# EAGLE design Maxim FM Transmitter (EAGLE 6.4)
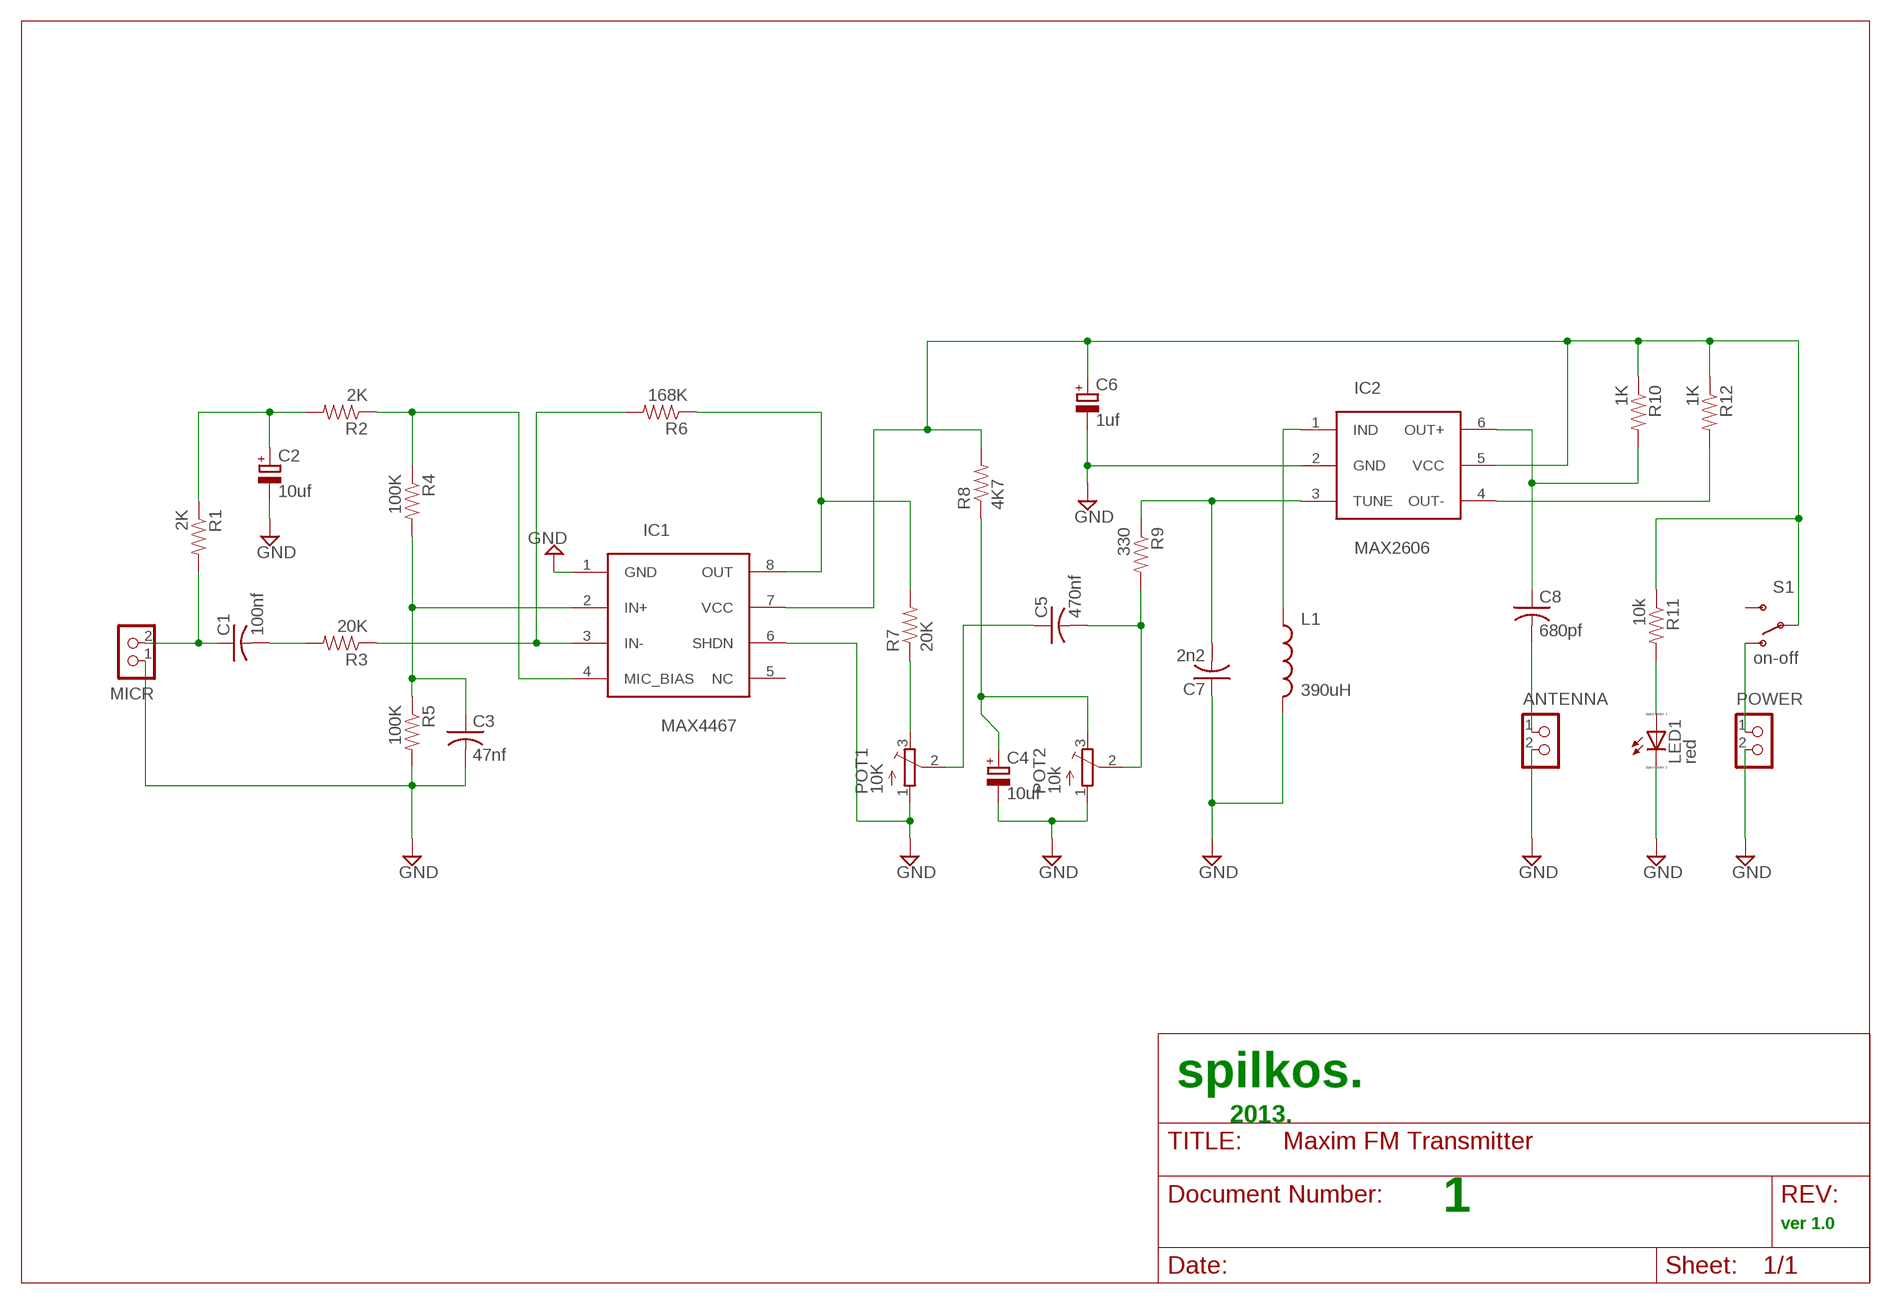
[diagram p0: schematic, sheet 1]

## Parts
ANTENNA  CON_HEADER_1X02-PTH  [M1X2]
C1  100nf  C-USC0805  [C0805]
C2  10uf  CPOL-EUSANYO_SMD_A5  [SANYO-OSCON_SMD_A5]
C3  47nf  C-USC0805  [C0805]
C4  10uf  CPOL-EUSANYO_SMD_A5  [SANYO-OSCON_SMD_A5]
C5  470nf  C-USC0805  [C0805]
C6  1uf  CPOL-EUSANYO_SMD_A5  [SANYO-OSCON_SMD_A5]
C7  2n2  C-USC0805  [C0805]
C8  680pf  C-USC0805  [C0805]
IC1  MAX4467  MAX4467-SOT-23-8L  [MAX4467-SOT-23-8L]
IC2  MAX2606  MAX2606-SOT-23-6L  [MAX2606-SOT-23-6L]
L1  390uH  INDUCTOR0805  [0805]
LED1  red  LED_ESML0603  [LED_SML0603]
MICR  micr  CON_HEADER_1X02-PTH  [M1X2]
POT1  10K  TRIMPOTTC33X  [TC33X]
POT2  10k  TRIMPOTTC33X  [TC33X]
POWER  power  CON_HEADER_1X02-PTH  [M1X2]
R1  2K  RESISTOR0805-RES  [0805]
R2  2K  RESISTOR0805-RES  [0805]
R3  20K  RESISTOR0805-RES  [0805]
R4  100K  RESISTOR0805-RES  [0805]
R5  100K  RESISTOR0805-RES  [0805]
R6  168K  RESISTOR0805-RES  [0805]
R7  20K  RESISTOR0805-RES  [0805]
R8  4K7  RESISTOR0805-RES  [0805]
R9  330  RESISTOR0805-RES  [0805]
R10  1K  RESISTOR0805-RES  [0805]
R11  10k  RESISTOR0805-RES  [0805]
R12  1K  RESISTOR0805-RES  [0805]
S1  on-off  SWITCH-SPDTSMD2  [SWITCH-SPDT-SMD]

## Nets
GND: ANTENNA.2 C2.- C3.2 C4.- C6.- C7.1 IC1.1(GND) IC1.6(SHDN) IC2.2(GND) L1.2 LED1.C MICR.1 POT1.1(A) POT2.1(A) POWER.2 R5.2
N$1: C1.1 MICR.2 R1.2
N$2: C1.2 R3.2
N$3: IC1.3(IN-) R3.1 R6.2
N$4: POT1.3(E) R7.1
N$5: C2.+ R1.1 R2.2
N$6: IC1.4(MIC_BIAS) R2.1 R4.1
N$7: C3.1 IC1.2(IN+) R4.2 R5.1
N$8: IC1.8(OUT) R6.1 R7.2
N$9: C4.+ POT2.3(E) R8.1
N$10: LED1.A R11.2
N$11: C5.1 POT1.2(S)
N$12: C5.2 POT2.2(S) R9.2
N$13: C7.2 IC2.3(TUNE) R9.1
N$14: IC2.1(IND) L1.1
N$15: IC2.4(OUT-) R12.2
N$16: ANTENNA.1 C8.2
N$17: C8.1 IC2.6(OUT+) R10.2
N$18: POWER.1 S1.1(O)
POWER: C6.+ IC1.7(VCC) IC2.5(VCC) R8.2 R10.1 R11.1 R12.1 S1.2(P)
Unconnected: IC1.5(NC) S1.3(S)

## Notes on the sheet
- spilkos.
- 2013.
- 1
- ver 1.0

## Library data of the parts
ANTENNA MICR POWER = dp_devices:CON_HEADER_1X02
C1 C3 C5 C7 C8 = adafruit:C-US: CAPACITOR, American symbol
C2 C4 C6 = rcl:CPOL-EU: POLARIZED CAPACITOR, European symbol
IC1 = MAX4467:MAX4467-SOT-23-8L
IC2 = MAX2606:MAX2606-SOT-23-6L
L1 = SparkFun-Passives:INDUCTOR: Inductors
LED1 = eagle-ltspice:LED_E: LED; SPICEMODEL: NONE; SPICEPREFIX: D; SPICETYPE: diode
POT1 POT2 = adafruit:TRIMPOT: SMT trimmer potentiometer part number TC33X http://www.ladyada.net/library/eagle
R1-R12 = SparkFun-Passives:RESISTOR: Resistor
S1 = SparkFun-Electromechanical:SWITCH-SPDT: SPDT Switch Simple slide switch, Spark Fun Electronics SKU : COM-00102 DPDT SMT slide switch, AYZ0202, SWCH-08179

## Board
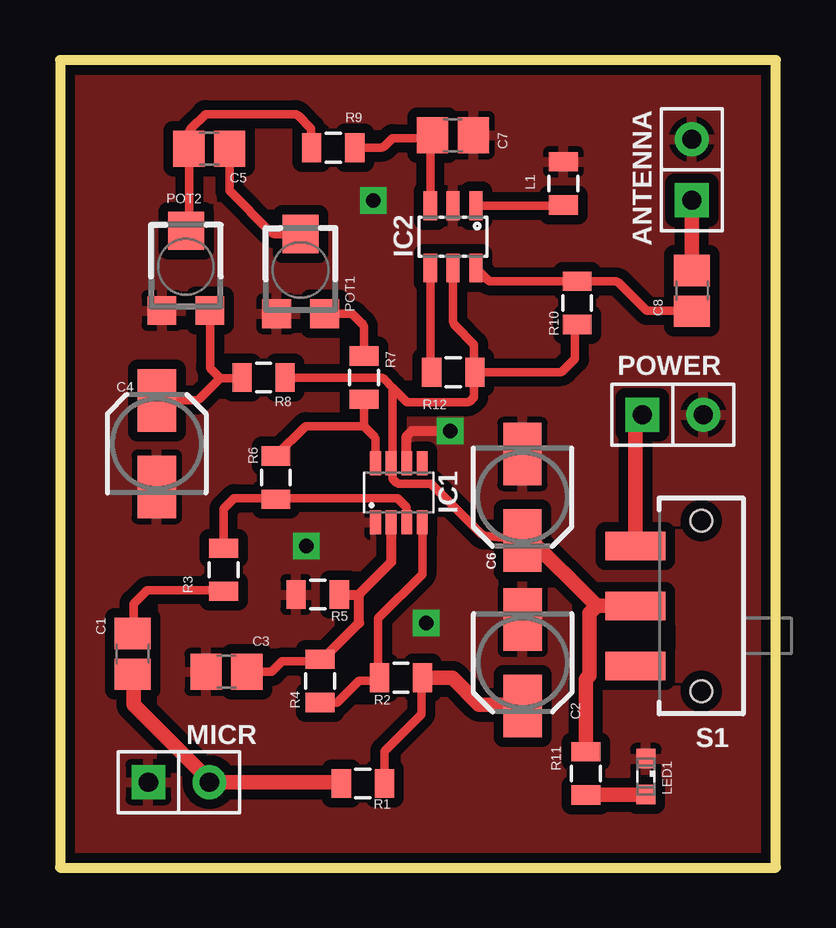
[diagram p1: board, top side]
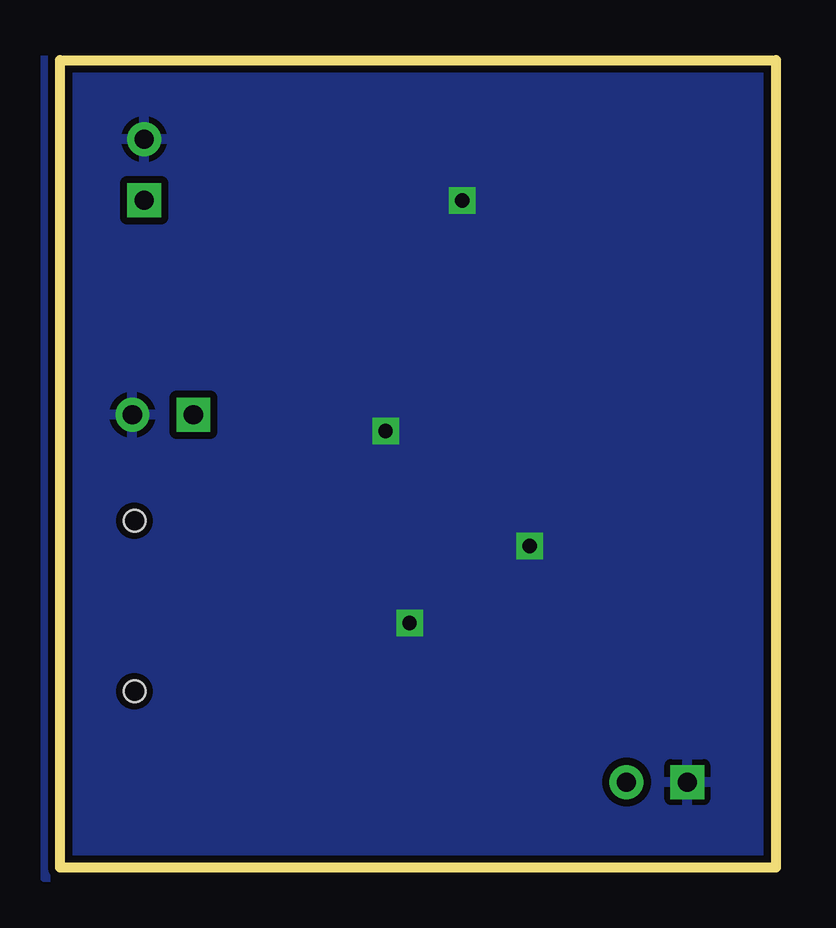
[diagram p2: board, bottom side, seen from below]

Size 29.84 x 33.66 mm. Coordinates in mm from the lower left corner, seen from the top.
Outline: 29.84,33.66 0,33.66 0,0 29.84,0 29.84,33.66
Copper layers (1*16): Top 0.035mm / dielectric 1.5mm / Bottom 0.035mm
Design rules "SparkFun": minimum track width 8mil, minimum drill 20mil, track to track 8mil, track to pad 8mil, pad to pad 8mil, via to via 8mil, smd to smd 8mil, copper to edge 10mil, drill to drill 8mil, minimum pad ring 12mil, minimum via ring 10mil, stop-mask expansion 4mil, vias tented up to drill 25mil, thermal gap 10mil
tRestrict: area 22.3,9.2 to 25.3,10; area 12.3,7.2 to 13.1,10.2; area 10.1,16 to 12.5,17.8

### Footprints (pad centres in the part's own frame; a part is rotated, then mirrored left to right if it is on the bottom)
M1X2 = drill 0.8 square: 1 -1.27,0 | drill 0.8: 2 1.27,0
C0805 = smd 1.3 x 1.5: 1 -0.85,0; 2 0.85,0
SANYO-OSCON_SMD_A5 = smd 2.6 x 1.6: + 1.8,0; - -1.8,0
MAX4467-SOT-23-8L = smd 1 x 0.45: 1 -1.225,0.975; 2 -1.225,0.325; 3 -1.225,-0.325; 4 -1.225,-0.975; 5 1.225,-0.975; 6 1.225,-0.325; 7 1.225,0.325; 8 1.225,0.975
MAX2606-SOT-23-6L = smd 1.2 x 0.55: 1 -1.3,0.95; 2 -1.3,0; 3 -1.3,-0.95; 4 1.3,-0.95; 5 1.3,0; 6 1.3,0.95
0805 = smd 0.8 x 1.2: 1 -0.9,0; 2 0.9,0
LED_SML0603 = smd 0.8 x 0.8: A 0.75,0; C -0.75,0
TC33X = smd 1.2 x 1.2: 1 -1,-1.825; 3 1,-1.825 | smd 1.5 x 1.6: 2 0,1.5
SWITCH-SPDT-SMD = smd 1.2 x 2.5: 1 -2.5,-2.75; 2 0,-2.75; 3 2.5,-2.75 | hole 0.9: -3.55,0; 3.55,0

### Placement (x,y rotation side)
ANTENNA  26.34,29.08 90 top
C1  3.03,8.91 90 top
C2  19.29,8.54 270 top
C3  6.95,8.16 180 top
C4  4.04,17.67 90 top
C5  6.23,29.96 180 top
C6  19.28,15.44 270 top
C7  16.38,30.52 180 top
C8  26.35,24.04 90 top
IC1  14.13,15.63 90 top
IC2  16.39,26.29 270 top
L1  20.99,28.51 90 top
LED1  24.43,3.8 270 top
MICR  4.96,3.57 0 top
POT1  10.03,24.9 0 top
POT2  5.25,25.04 0 top
POWER  25.55,18.88 0 top
R1  12.63,3.51 180 top
R2  14.22,7.91 0 top
R3  6.82,12.42 270 top
R4  10.85,7.78 90 top
R5  10.74,11.38 180 top
R6  9,16.26 270 top
R7  12.67,20.42 270 top
R8  8.49,20.42 0 top
R9  11.39,30 180 top
R10  21.56,23.53 90 top
R11  21.93,3.93 270 top
R12  16.4,20.65 180 top
S1  26.74,10.91 270 top

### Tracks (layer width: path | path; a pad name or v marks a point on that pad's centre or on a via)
GND  (via drill 0.6)
  Top 0.406: IC1.6 14.46,17.99 14.67,18.2 v16.27,18.2
  other vias: 13.07,27.8 15.27,10.2 10.27,13.4
  pour Top (isolate 0.406): 0,33.97 30.16,33.97 30.16,-0.32 0,-0.32
  pour Bottom (isolate 0.305): -0.33,34 30.22,34 30.47,33.75 30.47,-0.4 -0.08,-0.4 -0.33,-0.15
N$1
  Top 0.61: R1.2 11.67,3.57 MICR.2 6.23,3.64 3.07,6.8 3.07,8.02 C1.1
N$2
  Top 0.35: R3.2 6.78,11.56 3.63,11.56 3.07,11 3.07,9.79 C1.2
N$3
  Top 0.35: IC1.3 14.46,15.01 14.07,15.4 9.04,15.4 R6.2 8.96,15.4 7.27,15.4 6.82,14.95 R3.1
N$4
  Top 0.35: R7.1 12.67,22.49 arc45 12.6,22.67 12.26,23 arc45 12.09,23.08 POT1.3
N$5
  Top 0.35: R1.1 13.53,4.86 15.07,6.4 15.07,7.86 R2.2
  Top 0.61: R2.2 16.36,7.91 17.47,6.8 18.83,6.8 C2.+
N$6
  Top 0.35: IC1.4 15.11,12.24 13.27,10.4 13.27,7.96 R2.1 13.21,7.8 12.47,7.8 11.55,6.88 R4.1
N$7
  Top 0.35: 10.84,8.69 arc45 R4.2 | 10.75,8.72 arc-45 R4.2 | C3.1 8.83,8.16 9.27,8.6 10.76,8.6 R4.2
  Top 0.406: IC1.2 13.81,12.74 12.45,11.38 | R5.1 12.45,11.38 | R4.2 10.95,8.68 12.47,10.2 12.47,11.36 12.45,11.38
N$8
  Top 0.35: IC1.8 13.16,17.81 arc45 13.08,17.99 12.67,18.4 | 12.67,18.4 R7.2 arc-45 R7.2 | R6.1 10.24,18.4 12.67,18.4
N$9
  Top 0.35: POT2.3 6.25,20.93 arc45 6.32,20.75 6.67,20.4 | 6.67,20.4 7.53,20.4 arc45 R8.1 | C4.+ 5.63,19.47 arc45 5.81,19.54 6.67,20.4
N$10
  Top 0.61: R11.2 24.41,3.03 LED1.A
N$11
  Top 0.35: POT1.2 8.97,26.4 arc-45 8.79,26.48 7.07,28.2 7.07,29.94 arc-45 C5.1
N$12
  Top 0.35: POT2.2 5.3,26.79 arc45 5.38,26.97 C5.2 5.38,30.6 arc-45 5.45,30.78 6.07,31.4 9.76,31.4 arc-45 9.94,31.33 10.47,30.8 10.47,30.05 arc45 R9.2
N$13
  Top 0.35: R9.1 13.37,30 arc45 13.55,30.08 13.87,30.4 15.3,30.4 arc45 15.48,30.47 C7.2 15.51,30.5 arc45 15.44,30.32 IC2.3
N$14
  Top 0.35: IC2.1 20.97,27.59 L1.1
N$15
  Top 0.35: IC2.4 15.44,20.79 arc45 R12.2
N$16
  Top 0.61: C8.2 26.35,27.78 arc45 ANTENNA.1
N$17
  Top 0.35: IC2.6 17.82,24.5 arc45 18,24.43 R10.2 23.13,24.43 arc-45 23.31,24.36 24.47,23.2 26.32,23.2 arc-45 C8.1
N$18
  Top 0.61: POWER.1 24.24,18.88 arc90 23.99,18.62 S1.1
POWER
  Top 0.35: R12.1 20.81,20.65 arc45 20.99,20.72 21.47,21.2 21.47,22.43 arc-45 21.54,22.61 R10.1 | IC2.5 16.39,22.79 arc45 16.46,22.61 17.27,21.8 17.27,20.71 arc45 R12.1 | C6.+ 17.73,13.84 arc-45 17.55,13.91 15.47,16 14.17,16 arc-45 14,16.07 13.87,16.2 13.87,16.7 arc45 IC1.7 arc45 13.87,17 13.87,20 | R8.2 13.34,20.42 arc-45 13.52,20.35 13.87,20 | 13.87,20 14.47,19.4 16.96,19.4 arc45 17.14,19.47 17.27,19.6 17.27,20.58 arc-45 R12.1
  Top 0.61: S1.2 22.38,10.91 | 22.38,10.91 22.07,10.6 22.07,8 21.93,7.86 R11.1 | C6.+ 19.44,13.84 22.38,10.91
